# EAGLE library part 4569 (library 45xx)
Programmable dual 4 bit binary/BCD down COUNTER
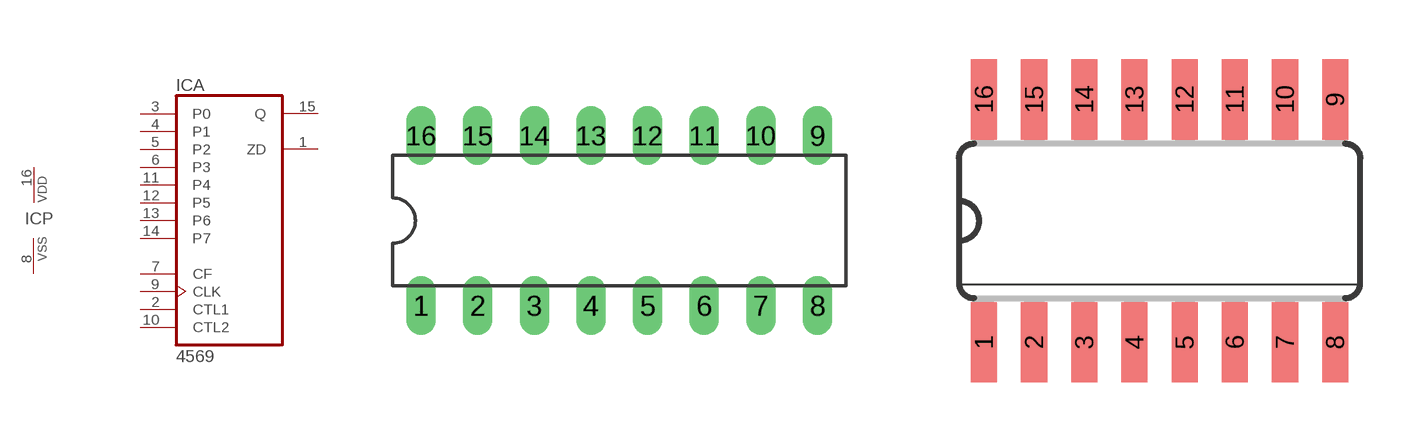
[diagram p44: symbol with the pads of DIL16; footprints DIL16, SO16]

Designator prefix IC; gates A=4569 P=PWRN

## 4569N  [DIL16]
1  A:ZD  out
2  A:CTL1  in
3  A:P0  in
4  A:P1  in
5  A:P2  in
6  A:P3  in
7  A:CF  in
8  P:VSS  pwr
9  A:CLK  in
10  A:CTL2  in
11  A:P4  in
12  A:P5  in
13  A:P6  in
14  A:P7  in
15  A:Q  out
16  P:VDD  pwr

## 4569D  [SO16]
Pads as for DIL16

## Footprint DIL16 (pad centres in mm)
Dual In Line Package
drill 0.813 long: 1 -8.89,-3.81; 2 -6.35,-3.81; 3 -3.81,-3.81; 4 -1.27,-3.81; 5 1.27,-3.81; 6 3.81,-3.81; 7 6.35,-3.81; 8 8.89,-3.81; 9 8.89,3.81; 10 6.35,3.81; 11 3.81,3.81; 12 1.27,3.81; 13 -1.27,3.81; 14 -3.81,3.81; 15 -6.35,3.81; 16 -8.89,3.81

## Footprint SO16 (pad centres in mm)
Small Outline package 150 mil
smd 0.66 x 2.032: 1 -4.445,-3.073; 2 -3.175,-3.073; 3 -1.905,-3.073; 4 -0.635,-3.073; 5 0.635,-3.073; 6 1.905,-3.073; 7 3.175,-3.073; 8 4.445,-3.073; 9 4.445,3.073; 10 3.175,3.073; 11 1.905,3.073; 12 0.635,3.073; 13 -0.635,3.073; 14 -1.905,3.073; 15 -3.175,3.073; 16 -4.445,3.073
